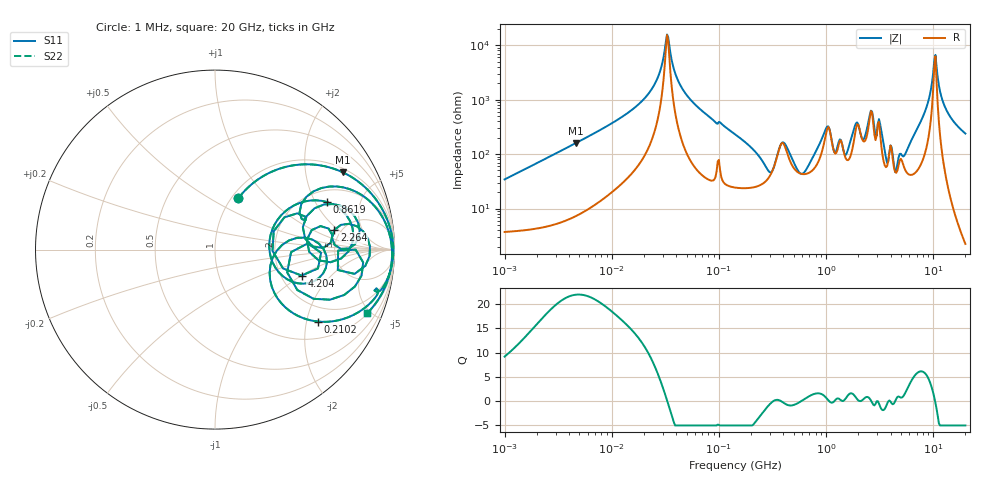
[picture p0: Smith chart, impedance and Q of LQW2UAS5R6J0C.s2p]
!Murata Part Number: LQW2UAS5R6J0C
!These Parameters are Measured in Series Mode Connection
!  o--[Z]--o
!Port1  Port2
!  o-------o
!Freq. Start=1[MHz] Stop=20[GHz], 401[Steps]
# Hz S RI R 50
!Freq.(Hz) S11(Real) S11(Imag) S21(Real) S21(Imag) S12(Real) S12(Imag) S22(Real) S22(Imag)
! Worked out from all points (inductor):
!   401 points, 1 MHz to 20 GHz, reference 50 ohm
!   read as one part in series: L = 5.41 uH near 1.051 MHz
!   highest Q = 21.9 at 4.642 MHz (marker M1), where L = 5.48 uH
!   self-resonance near 32.82 MHz
!   S11 on the Smith chart (normalised r, x): 1 MHz: 1.07, +0.68; 210.2 MHz: 1.49, -2.35; 861.9 MHz: 2.56, +2.51; 2.264 GHz: 4.39, +1.79; 4.204 GHz: 2.58, -1.00; 20 GHz: 1.04, -4.77
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1000000  0.1299 0.2861  0.8701 -0.2861  0.8701 -0.2861  0.1299 0.2861
4641514  0.7107 0.4312  0.2893 -0.4312  0.2893 -0.4312  0.7107 0.4312
5253183  0.7581 0.406  0.2419 -0.406  0.2419 -0.406  0.7581 0.406
1.640745e7  0.9716 0.1341  0.0284 -0.1341  0.0284 -0.1341  0.9716 0.1341
2.759593e7  0.9922 0.0333  0.0078 -0.0333  0.0078 -0.0333  0.9922 0.0333
3.364075e7  0.9938 -0.00347  0.00618 0.00347  0.00618 0.00347  0.9938 -0.00347
4.999273e7  0.9866 -0.0801  0.0134 0.0801  0.0134 0.0801  0.9866 -0.0801
1.414214e8  0.8184 -0.3363  0.1816 0.3363  0.1816 0.3363  0.8184 -0.3363
2.10163e8  0.5754 -0.4009  0.4246 0.4009  0.4246 0.4009  0.5754 -0.4009
3.046806e8  0.3086 -0.0876  0.6914 0.0876  0.6914 0.0876  0.3086 -0.0876
4.876899e8  0.4314 -0.1796  0.5686 0.1796  0.5686 0.1796  0.4314 -0.1796
7.429123e8  0.442 0.2471  0.558 -0.2471  0.558 -0.2471  0.442 0.2471
8.618922e8  0.6244 0.2646  0.3756 -0.2646  0.3756 -0.2646  0.6244 0.2646
1.1317e9  0.6437 -0.0705  0.3563 0.0705  0.3563 0.0705  0.6437 -0.0705
2.263619e9  0.6657 0.1108  0.3343 -0.1108  0.3343 -0.1108  0.6657 0.1108
2.626146e9  0.8632 0.0173  0.1368 -0.0173  0.1368 -0.0173  0.8632 0.0173
3.902654e9  0.5169 0.0347  0.4831 -0.0347  0.4831 -0.0347  0.5169 0.0347
4.203565e9  0.4823 -0.1446  0.5177 0.1446  0.5177 0.1446  0.4823 -0.1446
7.24727e9  0.8741 0.2581  0.1259 -0.2581  0.1259 -0.2581  0.8741 0.2581
1.050662e10  0.986 -0.00495  0.014 0.00495  0.014 0.00495  0.986 -0.00495
1.312914e10  0.9711 -0.1417  0.0289 0.1417  0.0289 0.1417  0.9711 -0.1417
2e10  0.8481 -0.3543  0.1519 0.3543  0.1519 0.3543  0.8481 -0.3543
